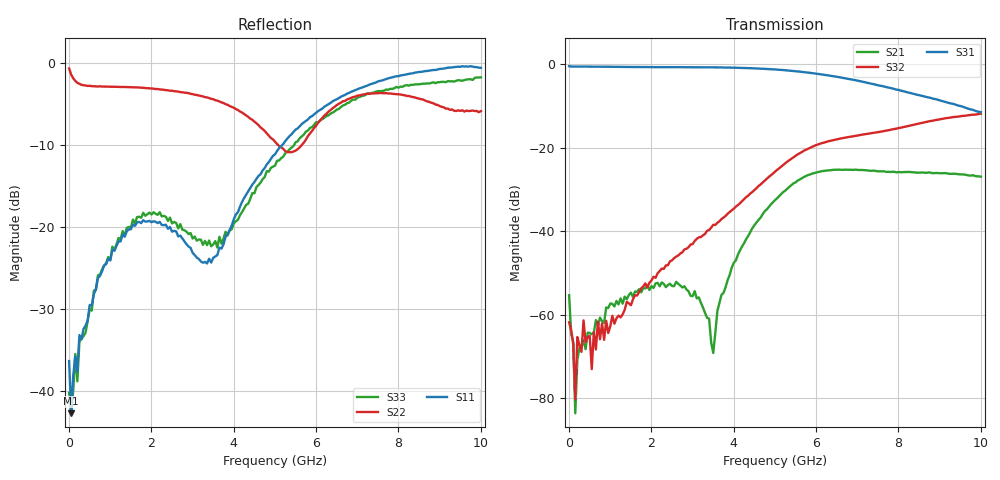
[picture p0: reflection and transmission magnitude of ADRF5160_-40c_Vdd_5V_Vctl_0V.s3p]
! Device:  ADRF5160
! Description: Silicon SPDT Switch
! Frequency:  0.7 -  4 GHz
! Ports:
!	RFc	= Port 1
!	RF1	= Port 2
!  RF2  = Port 3
! Vdd:  5 Volt
! Control:  0 Volt
! Data:  Data was collected using a calibrated 4 port network analyzer and de-embedded using Agilent's AFR De-Embedding.
! Note:  Analog Devices supplies this data as a sample of measured data
!  for this product.  Your particular data for this product may vary.
!  Data was taken at -40 degrees C.
!S3P File: Measurements: <S11,S12,S13>,
!<S21,S22,S23>,
!<S31,S32,S33>:
# Hz S  dB  R 50
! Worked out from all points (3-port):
!   201 points, 10 MHz to 10 GHz, reference 50 ohm
!   strongest paths, dB at 10 MHz, 2.507 GHz, 5.005 GHz, 7.503 GHz, 10 GHz:
!     S31: -0.4, -0.6, -1.2, -5.0, -11.4
!     S32: -61.8, -47.0, -25.7, -16.3, -11.8
!     S21: -55.3, -53.1, -32.5, -25.6, -26.9
!   lowest |S11| = -42.8 dB at 59.95 MHz (marker M1), VSWR 1.01, Z = 50.3 - j0.681 ohm
!   |S11| at or under -10 dB: start of sweep to 5.174 GHz
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1e7  -36.38 17.1  -55.47 -40.9  -0.39 -0.7
     -55.34 -130.7  -0.61 -8.7  -61.64 149.1
     -0.40 -0.6  -61.83 -37.6  -40.28 -34.0
5.995e7  -42.77 -68.7  -64.53 -75.3  -0.48 -2.0
         -64.50 162.9  -1.36 -45.4  -65.95 157.2
         -0.48 -1.8  -63.76 179.1  -42.69 -63.4
1.5985e8  -35.80 -86.7  -75.31 71.2  -0.50 -4.5
          -83.65 15.5  -2.12 -94.2  -73.59 38.6
          -0.49 -4.5  -80.31 111.0  -35.52 -74.8
2.098e8  -37.68 -78.1  -69.95 108.8  -0.50 -5.7
         -70.83 151.2  -2.36 -110.1  -69.55 6.3
         -0.50 -5.7  -65.35 27.2  -38.86 -86.1
6.094e8  -28.20 -96.8  -62.09 74.8  -0.52 -16.3
         -64.42 88.5  -2.78 -162.9  -66.08 -97.0
         -0.52 -16.3  -64.10 -116.7  -27.78 -116.8
2.6074e9  -20.52 -170.6  -52.53 48.9  -0.65 -69.5
          -52.12 52.3  -3.42 136.9  -45.87 -176.7
          -0.65 -69.4  -46.08 -173.1  -19.50 -147.2
3.5065e9  -23.76 103.1  -67.13 -77.4  -0.69 -94.7
          -69.19 -60.1  -4.36 114.5  -38.64 170.8
          -0.69 -94.6  -38.46 168.6  -22.11 -134.2
5.005e9  -11.11 22.2  -32.47 140.5  -1.19 -140.5
         -32.54 140.8  -9.56 77.5  -25.73 129.1
         -1.19 -140.4  -25.69 128.9  -12.49 -134.8
7.3027e9  -2.57 -39.5  -25.48 2.1  -4.53 147.2
          -25.48 2.0  -3.70 73.5  -16.57 15.4
          -4.53 147.3  -16.55 15.4  -3.66 149.1
1e10  -0.53 -73.2  -26.79 -82.2  -11.44 84.0
      -26.90 -81.7  -5.82 -13.4  -11.80 -82.4
      -11.44 84.1  -11.79 -82.4  -1.70 60.7
